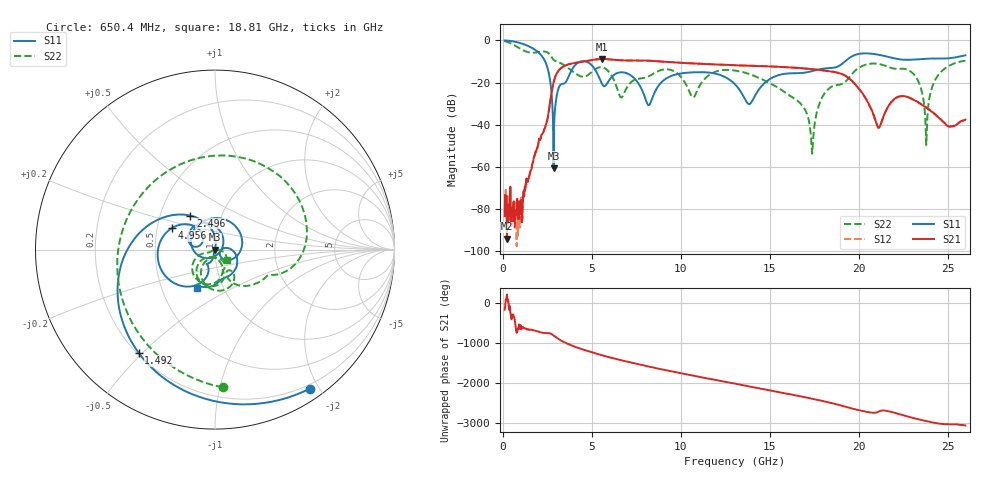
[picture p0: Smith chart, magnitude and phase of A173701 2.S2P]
!  2-Port S-parameters saved by WinCal
! VAR MeasName=S-Parameters (CALIBRATED_DATA) read from VNA (N5245A)
! VAR MeasDate=2017-6-7 10:28:35
! VAR NAME=A173701 2
! VAR FILENAME=A173701 2.S2P
! VAR DATE=2017-6-7 10:28:35
! VAR PHYS_PORTS=1,2
# Hz S DB R 50
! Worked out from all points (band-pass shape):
!   801 points, 100 MHz to 26 GHz, reference 50 ohm
!   highest |S21| = -8.79 dB at 5.571 GHz (marker M1); lowest = -94.3 dB at 229.5 MHz (marker M2)
!   |S21| within 3 dB of the highest: 3.553 GHz to 13.05 GHz (9.501 GHz wide, 114 % of centre); 13.10607 GHz to 13.12438 GHz (18.31 MHz wide, 0.14 % of centre)
!   lowest |S11| = -60.8 dB at 2.852 GHz (marker M3), VSWR 1.00, Z = 49.9 - j8.12e-05 ohm
!   |S11| at or under -10 dB: 2.378 GHz to 4.372 GHz (1.994 GHz wide, 59.1 % of centre); 4.662 GHz to 19.23 GHz (14.57 GHz wide, 122 % of centre)
!   |S22| runs from -53.8 to -0.2 dB; largest |S21 - S12| = 0.004
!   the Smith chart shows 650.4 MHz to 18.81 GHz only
!   S11 on the Smith chart (normalised r, x): 650.4 MHz: 0.15, -1.88; 1.492 GHz: 0.21, -0.49; 2.496 GHz: 0.71, +0.28; 4.956 GHz: 0.60, +0.16; 18.81 GHz: 0.75, -0.34
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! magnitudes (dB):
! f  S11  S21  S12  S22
! 100 MHz  0.0  -83.5  -78.9  -0.2
! 229.5 MHz  -0.1  -94.3  -87.5  -0.6
! 650.4 MHz  -0.6  -88.9  -84.7  -2.3
! 1.492 GHz  -2.9  -64.3  -64.2  -5.7
! 2.496 GHz  -12.6  -37.9  -37.9  -5.6
! 2.852 GHz  -60.8  -20.0  -20.0  -9.2
! 4.438 GHz  -9.9  -10.2  -10.2  -17.2
! 4.956 GHz  -11.5  -9.4  -9.4  -15.3
! 5.571 GHz  -20.6  -8.8  -8.8  -12.8
! 6.672 GHz  -15.1  -9.4  -9.5  -27.1
! 8.744 GHz  -21.6  -9.9  -9.9  -14.6
! 10.69 GHz  -15.2  -10.9  -11.0  -27.1
! 13.05 GHz  -20.8  -11.8  -11.8  -14.3
! 16.61 GHz  -15.5  -13.1  -13.0  -29.0
! 17.39 GHz  -14.5  -13.7  -13.6  -53.8
! 18.81 GHz  -12.5  -15.3  -15.2  -21.2
! 21.11 GHz  -6.8  -41.5  -41.5  -11.2
! 21.69 GHz  -7.9  -30.9  -31.1  -12.7
! 23.15 GHz  -9.1  -28.5  -28.4  -16.6
! 23.8 GHz  -8.7  -31.9  -31.8  -49.7
! 24.45 GHz  -8.6  -36.3  -36.1  -16.8
! 26 GHz  -7.1  -37.6  -37.5  -9.7
